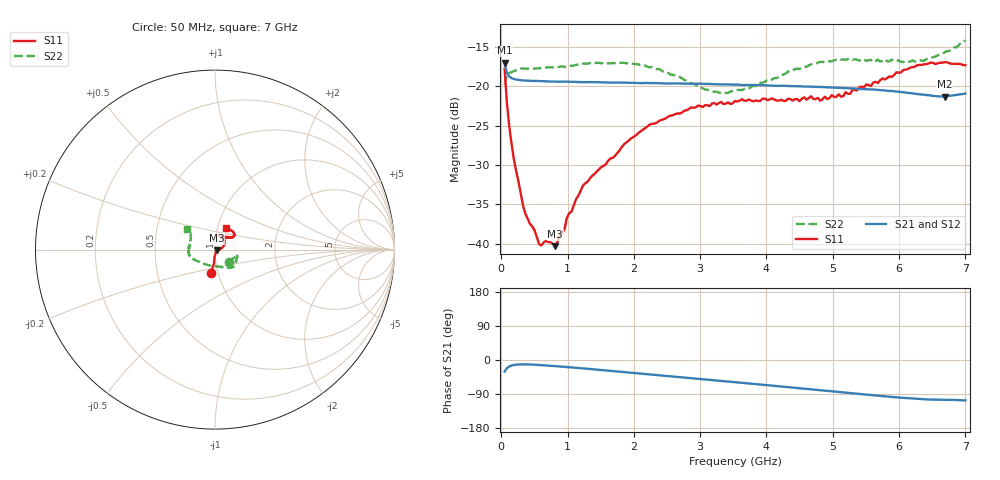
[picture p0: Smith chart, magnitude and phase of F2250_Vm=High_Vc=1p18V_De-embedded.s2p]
! Integrated Device Technology
! Corporate Headquarters
! 6024 Silver Creek Valley Road
! San Jose, CA 95138  USA
! Phone:  1-408-284-8200
! Toll Free:  1-800-223-1366
! Webpage:  http://www.idt.com/
! Timing and RF Division
! 515 Groton Road, Suite 102
! Westford, MA 01886-6024
! Device:  F2250
! Description: Voltage Variable RF Attenuator
! Frequency:  50.0 -  6000.00 MHz
! Package:  3x3 mm Thin QFN Plastic Package: 16 pin
! Ports:  2 RF, 3 DC
!  Pin  1  = GND
!  Pin  2  = NC
!  Pin  3  = RF1  = Port 1
!  Pin  4  = NC
!  Pin  5  = GND
!  Pin  6  = GND
!  Pin  7  = GND
!  Pin  8  = GND
!  Pin  9  = NC
!  Pin 10  = RF2  = Port 2
!  Pin 11  = NC
!  Pin 12  = GND
!  Pin 13  = GND
!  Pin 14  = VCNTRL
!  Pin 15  = VDD
!  Pin 16  = VMODE
! Vcntrl:  1.180 Volts
! Vmode:  +3.300 Volts
! Vdd:  +3.30  Volts
! Current:  1.330 mA
! Data:  The device was measured on a the F2250 evaluation board which has
!  individual transmission lines to the RF pins.  Data was collected
!  using a calibrated network analyzer.  The evaluation board was
!  de-embedded using a TRL calibration technique.
!  The reference plane is the edge of the package pin.
! Misc:  SN 10
!  Action Tracker AT0258
! Date Measured:  2014-11-26
! Date:  2015-10-15  MJV
! Note:
!  Integrated Device Technology supplies this data as a sample of measured
!  data at the package pin for this product.  Your particular data for this
!  product may vary.
!  Data was taken at 25 degrees C.
!  Integrated Device Technology reserves the right to change this data at anytime.
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# GHz S dB R 50
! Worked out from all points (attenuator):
!   201 points, 50 MHz to 7 GHz, reference 50 ohm
!   highest |S21| = -17.00 dB at 50 MHz (marker M1); lowest = -21.3 dB at 6.687 GHz (marker M2)
!   lowest |S11| = -40.3 dB at 814.5 MHz (marker M3), VSWR 1.02, Z = 50.9 - j0.345 ohm
!   |S11| at or under -10 dB: start of sweep to end of sweep
!   |S22| runs from -20.9 to -14.2 dB; largest |S21 - S12| = 0.00041
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0.05  -17.73 -100.1  -17.00 -30.5  -16.99 -30.4  -19.79 -42.3
0.08475  -22.10 -94.2  -18.31 -21.6  -18.30 -21.6  -18.54 -20.9
0.15425  -27.27 -93.7  -18.95 -14.6  -18.96 -14.6  -18.21 -13.0
0.189  -29.25 -91.7  -19.07 -13.2  -19.08 -13.2  -18.06 -12.5
0.328  -35.14 -78.7  -19.25 -11.5  -19.25 -11.5  -17.73 -12.8
0.57125  -40.05 -47.3  -19.33 -13.1  -19.32 -13.1  -17.71 -17.9
0.6755  -39.64 -42.4  -19.36 -14.3  -19.36 -14.3  -17.61 -20.1
0.8145  -40.30 -20.5  -19.39 -16.1  -19.39 -16.1  -17.59 -24.0
0.884  -38.81 -18.4  -19.40 -17.1  -19.39 -17.1  -17.52 -26.3
0.9535  -38.15 -23.6  -19.40 -18.0  -19.39 -18.1  -17.54 -27.6
0.98825  -36.73 -20.5  -19.41 -18.5  -19.41 -18.5  -17.48 -28.4
1.2315  -32.61 -3.6  -19.46 -22.1  -19.45 -22.1  -17.11 -33.5
1.857  -27.30 15.8  -19.54 -31.7  -19.52 -31.8  -17.02 -43.5
2.37825  -24.42 29.6  -19.62 -39.9  -19.62 -40.0  -17.79 -52.7
3.1775  -22.18 52.4  -19.72 -52.9  -19.70 -52.9  -20.66 -85.9
3.525  -21.87 63.1  -19.79 -58.6  -19.77 -58.6  -20.59 -110.0
4.7065  -21.61 67.8  -20.05 -78.1  -20.04 -78.1  -17.22 -160.2
5.15825  -21.26 51.2  -20.22 -85.5  -20.20 -85.6  -16.57 -169.3
5.85325  -18.73 36.3  -20.59 -96.8  -20.58 -97.0  -16.82 175.1
6.3745  -17.20 38.1  -21.06 -103.7  -21.08 -103.7  -16.77 157.4
6.68725  -16.93 45.7  -21.30 -104.9  -21.28 -105.1  -15.69 146.1
7  -17.33 62.0  -20.91 -106.7  -20.92 -106.8  -14.17 143.2
